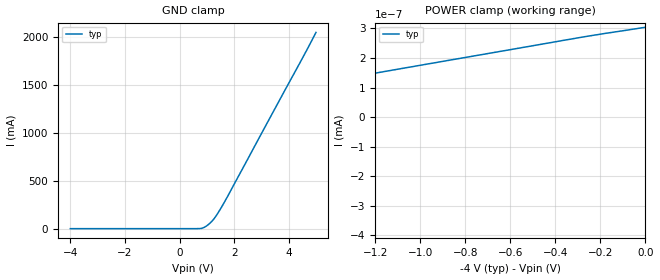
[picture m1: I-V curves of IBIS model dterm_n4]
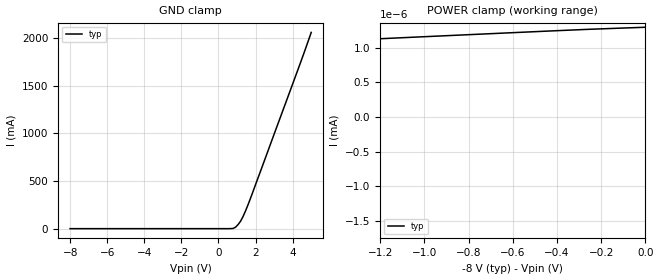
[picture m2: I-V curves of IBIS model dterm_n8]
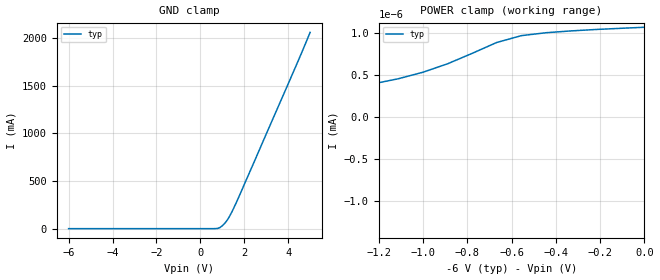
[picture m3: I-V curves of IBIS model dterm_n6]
|Texas Instruments Incorporated
|tmux4157n, 2:1x1 Negative switch
[IBIS Ver]   4.1
[File name]   tmux4157n.ibs
[Date]   02/02/21
[File Rev]   1.0
[Source]
| Texas Instruments Incorporated.
| ASC-INT-MPD
| 12500 TI Blvd
| Dallas, TX - 75243
[Notes]   Revision History:
| Rev 1.0: 02/02/21
| - Initial version of the model
| - Model generated from simulations in SPECTRE
| - C_comp although listed in numerical order of value are
|   obtained from varying PVT conditions. For PVT conditions for
|   each specific value refer the buffer description under
|   respective [Model]. IBIS model user is responsible for using
|   appropriate C_comp to simulate for Signal Integrity.
[Disclaimer]
| This model is designed as an aid for customers of Texas Instruments.
| TI and its licensors and suppliers make no warranties, either expressed
| or implied, with respect to this  model, including the warranties of
| merchantability or fitness for a particular purpose. The model is
| provided solely on an "as is" basis. The entire risk as to its quality
| and performance is with the customer.
| This model is subject to change without notice. Texas Instruments
| Incorporated is not responsible for updating this model.
[Copyright]
(C) Copyright 2021 Texas Instruments Incorporated.All rights reserved.
|  Component TMUX4157NPW 6-pin - PW package
|  Part # TMUX4157NPW
[Component]   TMUX4157NPW
[Manufacturer]  TI
[Package]
|   typ   min   max
R_pkg   0.05   0.05   0.05
L_pkg   1.0nH   1.0nH   1.0nH
C_pkg   0.2pF   0.2pF   0.2pF
[Pin]   signal_name   model_name   R_pin  L_pin  C_pin
   1   S2   sterm   NA   NA   NA
   2   VSS   power   NA   NA   NA
   3   S1   sterm   NA   NA   NA
   4   SEL   inbuf   NA   NA   NA
   5   GND   gnd   NA   NA   NA
   6   D   dterm   NA   NA   NA
[Series Switch Groups]
On 1 /
On 2 /
[Series Pin Mapping]  pin_2 model_name function_table_group
3 6 switch_n4 1
1 6 switch_n4 2
3 6 switch_n8 1
1 6 switch_n8 2
3 6 switch_n6 1
1 6 switch_n6 2
3 6 switch_n12 1
1 6 switch_n12 2
3 6 switch_n10 1
1 6 switch_n10 2
[Model Selector] dterm
dterm_n4 Use for operation at -4V
dterm_n8 Use for operation at -8V
dterm_n6 Use for operation at -6V
dterm_n12 Use for operation at -12V
dterm_n10 Use for operation at -10V
[Model Selector] sterm
sterm_n4 Use for operation at -4V
sterm_n8 Use for operation at -8V
sterm_n6 Use for operation at -6V
sterm_n12 Use for operation at -12V
sterm_n10 Use for operation at -10V
[Model Selector] inbuf
inbuf_n4 Use for operation at -4V
inbuf_n8 Use for operation at -8V
inbuf_n6 Use for operation at -6V
inbuf_n12 Use for operation at -12V
inbuf_n10 Use for operation at -10V
| switch_n4
[Model]   switch_n4
Model_type   Series_switch
|   typ   min   max
C_comp   1.457606e-11   NA   NA
[Voltage Range]   -4   NA   NA
[Temperature Range]   27   NA   NA
[On]
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[Off]
|   typ   min   max
[R Series]   10G   NA   NA
| switch_n8
[Model]   switch_n8
Model_type   Series_switch
|   typ   min   max
C_comp   1.457606e-11   NA   NA
[Voltage Range]   -8   NA   NA
[Temperature Range]   27   NA   NA
[On]
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[Off]
|   typ   min   max
[R Series]   10G   NA   NA
| switch_n6
[Model]   switch_n6
Model_type   Series_switch
|   typ   min   max
C_comp   1.457606e-11   NA   NA
[Voltage Range]   -6   NA   NA
[Temperature Range]   27   NA   NA
[On]
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[Off]
|   typ   min   max
[R Series]   10G   NA   NA
| switch_n12
[Model]   switch_n12
Model_type   Series_switch
|   typ   min   max
C_comp   1.008417e-11   NA   NA
[Voltage Range]   -12   NA   NA
[Temperature Range]   27   NA   NA
[On]
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[Off]
|   typ   min   max
[R Series]   10G   NA   NA
| switch_n10
[Model]   switch_n10
Model_type   Series_switch
|   typ   min   max
C_comp   1.457606e-11   NA   NA
[Voltage Range]   -10   NA   NA
[Temperature Range]   27   NA   NA
[On]
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[Off]
|   typ   min   max
[R Series]   10G   NA   NA
| Models and submodels in the file (20): dterm_n4 (Terminator), dterm_n8 (Terminator), dterm_n6 (Terminator), dterm_n12 (Terminator), dterm_n10 (Terminator), switch_n4 (Series_switch), switch_n8 (Series_switch), switch_n6 (Series_switch), switch_n12 (Series_switch), switch_n10 (Series_switch), sterm_n4 (Terminator), sterm_n8 (Terminator), sterm_n6 (Terminator), sterm_n12 (Terminator), sterm_n10 (Terminator), inbuf_n4 (Input), inbuf_n8 (Input), inbuf_n6 (Input), inbuf_n12 (Input), inbuf_n10 (Input)
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| dterm_n4
[Model]   dterm_n4
Model_type   Terminator
|   typ   min   max
C_comp   1.457606e-11   NA   NA
[Voltage Range]   -4   NA   NA
[Temperature Range]   27   NA   NA
[Power Clamp Reference]   -4   NA   NA
[GND Clamp Reference]   0   NA   NA
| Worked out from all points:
|   POWER clamp passes 1 mA (typ) near -4.73 V on its own axis
[GND Clamp]
|   Voltage   I(typ)   I(min)   I(max)
-4V       -252.6pA   NA         NA
727.3mV   925uA      NA         NA
909.1mV   13.74mA    NA         NA
1.091V    50.9mA     NA         NA
1.182V    75.26mA    NA         NA
1.364V    143.5mA    NA         NA
1.727V    318.9mA    NA         NA
4.545V    1.803A     NA         NA
5V        2.05A      NA         NA
[POWER Clamp]
|   Voltage   I(typ)   I(min)   I(max)
-9V       -2.154A    NA         NA
-4.182V   -774.5pA   NA         NA
-4.091V   -282.7pA   NA         NA
-4V       -252.7pA   NA         NA
-2.727V   -64.1pA    NA         NA
-2V       39.59pA    NA         NA
-363.6mV  259.8pA    NA         NA
0V        304.1pA    NA         NA
| dterm_n8
[Model]   dterm_n8
Model_type   Terminator
|   typ   min   max
C_comp   1.457606e-11   NA   NA
[Voltage Range]   -8   NA   NA
[Temperature Range]   27   NA   NA
[Power Clamp Reference]   -8   NA   NA
[GND Clamp Reference]   0   NA   NA
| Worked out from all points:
|   POWER clamp passes 1 mA (typ) near -8.70 V on its own axis
[GND Clamp]
|   Voltage   I(typ)   I(min)   I(max)
-8V       -692.7pA   NA         NA
535.4mV   23.3uA     NA         NA
798mV     2.59mA     NA         NA
929.3mV   17mA       NA         NA
1.192V    78.44mA    NA         NA
1.323V    126.5mA    NA         NA
1.586V    247.5mA    NA         NA
4.343V    1.701A     NA         NA
5V        2.06A      NA         NA
[POWER Clamp]
|   Voltage   I(typ)   I(min)   I(max)
-13V      -2.156A    NA         NA
-8.273V   -11.25nA   NA         NA
-8.141V   -840.2pA   NA         NA
-8.01V    -694.9pA   NA         NA
-6.303V   -346.7pA   NA         NA
-3.545V   150.4pA    NA         NA
-3.283V   238.2pA    NA         NA
-3.02V    391pA      NA         NA
-2.889V   510.5pA    NA         NA
-2.626V   827.4pA    NA         NA
-2.495V   912.9pA    NA         NA
0V        1.298nA    NA         NA
| dterm_n6
[Model]   dterm_n6
Model_type   Terminator
|   typ   min   max
C_comp   1.457606e-11   NA   NA
[Voltage Range]   -6   NA   NA
[Temperature Range]   27   NA   NA
[Power Clamp Reference]   -6   NA   NA
[GND Clamp Reference]   0   NA   NA
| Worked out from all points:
|   POWER clamp passes 1 mA (typ) near -6.71 V on its own axis
[GND Clamp]
|   Voltage   I(typ)   I(min)   I(max)
-6V       -439.1pA   NA         NA
666.7mV   425uA      NA         NA
888.9mV   10.85mA    NA         NA
1V        30.3mA     NA         NA
1.222V    88.21mA    NA         NA
1.333V    130.7mA    NA         NA
1.667V    288.1mA    NA         NA
4.333V    1.696A     NA         NA
5V        2.06A      NA         NA
[POWER Clamp]
|   Voltage   I(typ)   I(min)   I(max)
-11V      -2.155A    NA         NA
-6.222V   -2.457nA   NA         NA
-6.111V   -495.9pA   NA         NA
-6V       -438.9pA   NA         NA
-1.556V   284pA      NA         NA
-1.333V   350.7pA    NA         NA
-1.111V   456.6pA    NA         NA
-888.9mV  634.7pA    NA         NA
-666.7mV  888.7pA    NA         NA
-555.6mV  970pA      NA         NA
-333.3mV  1.026nA    NA         NA
0V        1.07nA     NA         NA
